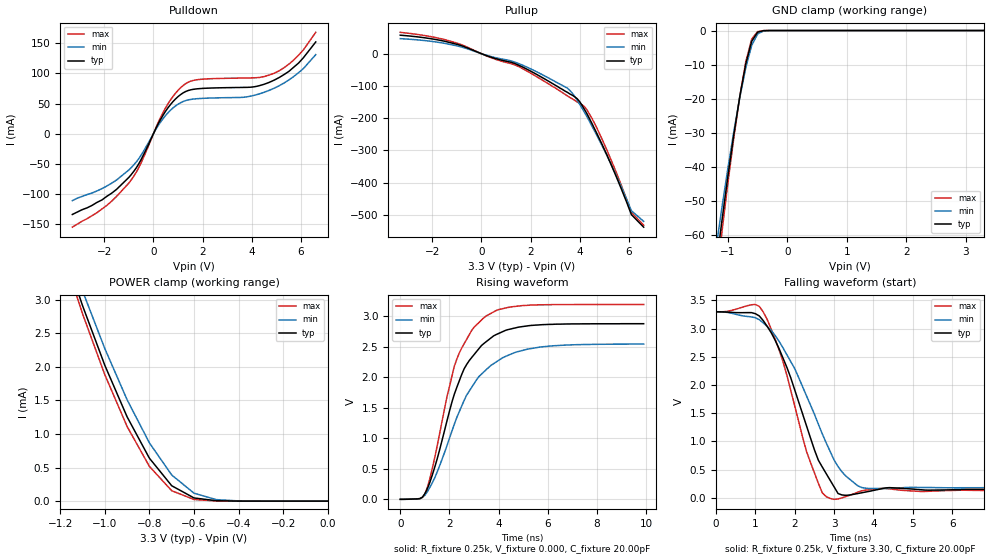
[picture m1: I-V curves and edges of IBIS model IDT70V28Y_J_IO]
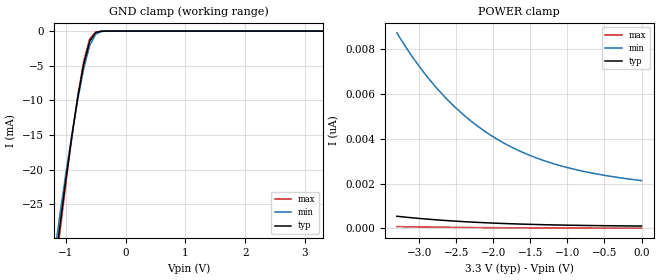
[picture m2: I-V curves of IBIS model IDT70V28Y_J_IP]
| IBIS file 70v9289y.ibs created by s2ibis2 version 1.1
| North Carolina State University Electronics Research Laboratory  1995
[IBIS ver]   2.1
[File name]   70v9289y.ibs
[File Rev]   1.0
[Date]   10/12/00
[Source]   Integrated Device Technology, Inc.
[Notes]   1.Temperatures: typ=25C, min=70C, max=0C 2.Ramp rates based on
   250 ohm load.
[Disclaimer] Integrated Device Technology, Inc. ("IDT") hereby grants the
   user of this IBIS model a non-exclusive, nontransferable
   license to use this IBIS model under the following terms. The
   user is granted this license only to use the IBIS model and is
   not granted rights to sell, copy (except as needed to run the
   IBIS model), rent, lease or sub-license the IBIS model in
   whole or in part, or in modified form to anyone. The User may
   modify the IBIS model to suit its specific applications, but
   rights to derivative works and such modifications shall belong
   to IDT. This IBIS model is provided on an AS IS" basis and IDT
   makes absolutely no warranty with respect to the information
   contained herein. IDT DISCLAIMS AND CUSTOMER WAIVES ALL
   WARRANTIES, EXPRESS AND IMPLIED, INCLUDING WARRANTIES OF
   MERCHANTABILITY AND FITNESS FOR A PARTICULAR PURPOSE. THE
   ENTIRE RISK AS TO QUALITY AND PERFORMANCE IS WITH THE USER
   ACCORDINGLY, IN NO EVENT SHALL IDT BE LIABLE FOR ANY DIRECT OR
   INDIRECT DAMAGES, WHETHER IN CONTRACT OR TORT, INCLUDING ANY
   LOST PROFITS OR OTHER INCIDENTAL, CONSEQUENTIAL, EXEMPLARY, OR
   PUNITIVE DAMAGES ARISING OUT OF THE USE OR APPLICATION OF THE
   IBIS model. Further, IDT reserves the right to make changes
   without notice to any product herein to improve reliability,
   function, or design. IDT does not convey any license under
   patent rights or any other intellectual property rights,
   including those of third parties. IDT is not obligated to
   provide maintenance or support for the licensed IBIS model.
[Copyright]   Copyright 2000, Integrated Device Technology, Inc. all rights
   reserved
|   Component 70v9289y
[Component]   70v9289y
[Manufacturer]   Integrated Device Technology
[Package]	 TQFP(PK128)
| variable   typ   min   max
R_pkg   10.00m   9.00m   11.00m
L_pkg   4.50nH   4.10nH   5.10nH
C_pkg   0.16pF   0.11pF   0.22pF
[Pin]  signal_name   model_name   R_pin   L_pin   C_pin
1   NC   NC
2   NC   NC
3   NC   NC
4   NC   NC
5   A9R   IDT70V28Y_J_IP
6   A8R   IDT70V28Y_J_IP
7   A7R   IDT70V28Y_J_IP
8   A6R   IDT70V28Y_J_IP
9   A5R   IDT70V28Y_J_IP
10   A4R   IDT70V28Y_J_IP
11   A3R   IDT70V28Y_J_IP
12   A2R   IDT70V28Y_J_IP
13   A1R   IDT70V28Y_J_IP
14   A0R   IDT70V28Y_J_IP
15   NC   NC
16   CNTENR#   IDT70V28Y_J_IP
17   CLKR   IDT70V28Y_J_IP
18   ADSR#   IDT70V28Y_J_IP
19   GND   GND
20   VCC   POWER
21   ADSL#   IDT70V28Y_J_IP
22   CLKL   IDT70V28Y_J_IP
23   CNTENL#   IDT70V28Y_J_IP
24   NC   NC
25   A0L   IDT70V28Y_J_IP
26   A1L   IDT70V28Y_J_IP
27   A2L   IDT70V28Y_J_IP
28   A3L   IDT70V28Y_J_IP
29   A4L   IDT70V28Y_J_IP
30   A5L   IDT70V28Y_J_IP
31   A6L   IDT70V28Y_J_IP
32   A7L   IDT70V28Y_J_IP
33   A8L   IDT70V28Y_J_IP
34   A9L   IDT70V28Y_J_IP
35   NC   NC
36   NC   NC
37   NC   NC
38   NC   NC
39   A10L   IDT70V28Y_J_IP
40   A11L   IDT70V28Y_J_IP
41   A12L   IDT70V28Y_J_IP
42   A13L   IDT70V28Y_J_IP
43   A14L   IDT70V28Y_J_IP
44   A15L   IDT70V28Y_J_IP
45   NC   NC
46   NC   NC
47   LBL#   IDT70V28Y_J_IP
48   UBL#   IDT70V28Y_J_IP
49   CE0L#   IDT70V28Y_J_IP
50   CE1L   IDT70V28Y_J_IP
51   CNTRRSTL#   IDT70V28Y_J_IP
52   VCC   POWER
53   GND   GND
54   RWL   IDT70V28Y_J_IP
55   OEL#   IDT70V28Y_J_IP
56   FTPLL   IDT70V28Y_J_IP
57   GND   GND
58   IO15L   IDT70V28Y_J_IO
59   IO14L   IDT70V28Y_J_IO
60   IO13L   IDT70V28Y_J_IO
61   IO12L   IDT70V28Y_J_IO
62   VCC   POWER
63   GND   GND
64   IO11L   IDT70V28Y_J_IO
65   IO10L   IDT70V28Y_J_IO
66   IO9L   IDT70V28Y_J_IO
67   VCC   POWER
68   NC   NC
69   IO8L   IDT70V28Y_J_IO
70   NC   NC
71   NC   NC
72   VCC   POWER
73   IO7L   IDT70V28Y_J_IO
74   IO6L   IDT70V28Y_J_IO
75   IO5L   IDT70V28Y_J_IO
76   IO4L   IDT70V28Y_J_IO
77   GND   GND
78   IO3L   IDT70V28Y_J_IO
79   IO2L   IDT70V28Y_J_IO
80   GND   GND
81   IO1L   IDT70V28Y_J_IO
82   IO0L   IDT70V28Y_J_IO
83   VCC   POWER
84   GND   GND
85   IO0R   IDT70V28Y_J_IO
86   IO1R   IDT70V28Y_J_IO
87   IO2R   IDT70V28Y_J_IO
88   VCC   POWER
89   IO3R   IDT70V28Y_J_IO
90   GND   GND
91   IO4R   IDT70V28Y_J_IO
92   IO5R   IDT70V28Y_J_IO
93   IO6R   IDT70V28Y_J_IO
94   VCC   POWER
95   IO7R   IDT70V28Y_J_IO
96   NC   NC
97   NC   NC
98   IO8R   IDT70V28Y_J_IO
99   NC   NC
100   GND   GND
101   IO9R   IDT70V28Y_J_IO
102   IO10R   IDT70V28Y_J_IO
103   IO11R   IDT70V28Y_J_IO
104   VCC   POWER
105   VCC   POWER
106   IO12R   IDT70V28Y_J_IO
107   IO13R   IDT70V28Y_J_IO
108   IO14R   IDT70V28Y_J_IO
109   IO15R   IDT70V28Y_J_IO
110   GND   GND
111   FTPLR   IDT70V28Y_J_IP
112   OER#   IDT70V28Y_J_IP
113   RWR   IDT70V28Y_J_IP
114   GND   GND
115   VCC   POWER
116   CNTRRSTR#   IDT70V28Y_J_IP
117   CE1R   IDT70V28Y_J_IP
118   CE0R#   IDT70V28Y_J_IP
119   UBR#   IDT70V28Y_J_IP
120   LBR#   IDT70V28Y_J_IP
121   NC   NC
122   NC   NC
123   A15R   IDT70V28Y_J_IP
124   A14R   IDT70V28Y_J_IP
125   A13R   IDT70V28Y_J_IP
126   A12R   IDT70V28Y_J_IP
127   A11R   IDT70V28Y_J_IP
128   A10R   IDT70V28Y_J_IP
| Models and submodels in the file (2): IDT70V28Y_J_IO (I/O), IDT70V28Y_J_IP (Input)
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| in   in   dummy_model
| oel  oel   dummy_model
|   Model IDT70V28Y_J_IO
[Model]   IDT70V28Y_J_IO
Model_type   I/O
Polarity   Non-Inverting
Enable   Active-High
Vinl =  0.800V
Vinh =  2.000V
Vmeas =  1.500V
C_comp   3.00pF   NA   NA
[Temperature Range]   25.00   70.00   0.000
[Voltage Range]   3.30V   3.00V   3.60V
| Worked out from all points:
|   slope of the pulldown table from 0 to 0.495 V, typ, clamps not added: 13.3 ohm
|   slope of the pullup table from 0 to 0.495 V, typ, clamps not added: 37.2 ohm
|   GND clamp passes 1 mA (typ) near -0.52 V on its own axis
|   POWER clamp passes 1 mA (typ) near -0.86 V on its own axis
|   rising waveform, R_fixture 0.25k, V_fixture 0.000, C_fixture 20.00pF: 20-80 % time 1.42ns typ, 1.7ns min, 1.23ns max; typ from 0 V to 2.88 V
|   falling waveform, R_fixture 0.25k, V_fixture 3.30, C_fixture 20.00pF: 20-80 % time 954ps typ, 1.22ns min, 749ps max; typ from 3.3 V to 0.148 V
[Pulldown]
| voltage   I(typ)   I(min)   I(max)
-3.3V     -134mA     -111mA     -155mA
-1.9V     -104mA     -86.9mA    -119mA
-1V       -72.45mA   -60.15mA   -81.9mA
-600mV    -50.19mA   -41.64mA   -56.6mA
500mV     37.63mA    30.47mA    43.27mA
1.2V      67.44mA    53.17mA    79.6mA
1.8V      74.41mA    58.03mA    89.56mA
3.8V      76.78mA    61.03mA    92.31mA
4.9V      88.52mA    75.19mA    100mA
5.7V      110mA      94.62mA    122mA
6.1V      126mA      108mA      139mA
6.6V      152mA      131mA      168mA
[Pullup]
| voltage   I(typ)   I(min)   I(max)
-3.3V     57.3mA     46.6mA     66.18mA
-1.5V     38.63mA    32.12mA    43.81mA
-800mV    24.35mA    20.41mA    27.47mA
500mV     -13.43mA   -11.1mA    -15.45mA
1.3V      -28.94mA   -24.66mA   -33.12mA
3.5V      -120mA     -107mA     -131mA
3.9V      -140mA     -145mA     -150mA
4.3V      -187mA     -196mA     -175mA
4.7V      -248mA     -254mA     -231mA
5.5V      -384mA     -380mA     -371mA
6.1V      -499mA     -487mA     -492mA
6.6V      -538mA     -520mA     -532mA
[GND_clamp]
| voltage   I(typ)   I(min)   I(max)
-3.3V     -467mA     -404mA     -524mA
-1.2V     -69.58mA   -64.01mA   -74.22mA
-1.1V     -55.82mA   -51.94mA   -59.11mA
-1V       -42.75mA   -40.45mA   -44.8mA
-900mV    -30.53mA   -29.64mA   -31.46mA
-800mV    -19.38mA   -19.68mA   -19.39mA
-700mV    -9.838mA   -10.96mA   -9.227mA
-600mV    -3.168mA   -4.369mA   -2.536mA
-500mV    -487uA     -999uA     -296uA
-400mV    -42.79uA   -132uA     -19.7uA
-300mV    -2.736uA   -13.26uA   -912nA
3.3V      192pA      371nA      23.19pA
[POWER_clamp]
| voltage   I(typ)   I(min)   I(max)
-3.3V     34.48mA    32.12mA    36.12mA
-1.2V     3.903mA    4.073mA    3.817mA
-1.1V     2.913mA    3.132mA    2.792mA
-1V       2.023mA    2.272mA    1.883mA
-900mV    1.255mA    1.509mA    1.111mA
-800mV    639uA      867uA      517uA
-700mV    229uA      389uA      155uA
-600mV    47.33uA    118uA      24.27uA
-500mV    5.976uA    22.31uA    2.392uA
-400mV    588nA      3.161uA    179nA
0V        192pA      3.664nA    26.38pA
[Ramp]
| variable   typ   min   max
dV/dt_r   1.73/0.43n   1.53/0.55n   1.92/0.33n
dV/dt_f   1.89/0.33n   1.70/0.44n   2.08/0.27n
R_load = 0.25k
[Rising Waveform]
R_fixture = 0.25k
V_fixture = 0.000
C_fixture = 20.00pF
R_dut = 100.00m
L_dut = 4.00nH
C_dut = 0.60pF
| time   V(typ)   V(min)   V(max)
0s        0V         0V         0V
800ps     12.02mV    11.87mV    12.31mV
1ns       91.19mV    65.8mV     85.41mV
1.4ns     523mV      350mV      680mV
2.2ns     1.724V     1.232V     2.182V
2.6ns     2.141V     1.623V     2.552V
3.4ns     2.554V     2.089V     2.977V
4.3ns     2.773V     2.346V     3.138V
5.2ns     2.845V     2.464V     3.181V
9.9ns     2.879V     2.545V     3.194V
[Falling Waveform]
R_fixture = 0.25k
V_fixture = 3.30
C_fixture = 20.00pF
R_dut = 100.00m
L_dut = 4.00nH
C_dut = 0.60pF
| time   V(typ)   V(min)   V(max)
0s        3.3V       3.3V       3.3V
1ns       3.266V     3.194V     3.429V
1.2ns     3.144V     3.103V     3.297V
1.7ns     2.482V     2.662V     2.42V
2.3ns     1.275V     1.808V     822mV
2.7ns     547mV      1.135V     90.16mV
2.9ns     312mV      822mV      -11.21mV
3.2ns     51.94mV    461mV      465uV
3.8ns     104mV      172mV      138mV
9.9ns     148mV      181mV      130mV
|   Model IDT70V28Y_J_IP
[Model]   IDT70V28Y_J_IP
Model_type   Input
Vinl =  0.800V
Vinh =  2.000V
Vmeas =  1.500V
C_comp   3.00pF   NA   NA
[Temperature Range]   25.00   70.00   0.000
[Voltage Range]   3.30V   3.00V   3.60V
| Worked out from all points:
|   GND clamp passes 1 mA (typ) near -0.56 V on its own axis
[GND_clamp]
| voltage   I(typ)   I(min)   I(max)
-3.3V     -208mA     -191mA     -218mA
-1.2V     -35.22mA   -32.9mA    -36.71mA
-1.1V     -28.21mA   -26.62mA   -29.22mA
-1V       -21.53mA   -20.65mA   -22.09mA
-900mV    -15.28mA   -15.03mA   -15.43mA
-800mV    -9.592mA   -9.878mA   -9.392mA
-700mV    -4.764mA   -5.402mA   -4.354mA
-600mV    -1.468mA   -2.085mA   -1.129mA
-500mV    -211uA     -452uA     -121uA
-400mV    -17.57uA   -57.18uA   -7.624uA
-300mV    -1.075uA   -5.508uA   -337nA
3.3V      109pA      2.266nA    13.01pA
[POWER_clamp]
| voltage   I(typ)   I(min)   I(max)
-3.3V     545pA      8.718nA    84.03pA
-3.2V     510pA      8.189nA    78.64pA
-3V       448pA      7.232nA    68.83pA
-2.7V     369pA      6.027nA    56.34pA
-2.4V     305pA      5.062nA    46.2pA
-2.2V     270pA      4.534nA    40.57pA
-2V       240pA      4.085nA    35.73pA
-1.8V     215pA      3.706nA    31.59pA
-1.6V     193pA      3.388nA    28.07pA
-1.2V     160pA      2.9nA      22.58pA
-700mV    132pA      2.491nA    17.95pA
0V        109pA      2.133nA    14.11pA
